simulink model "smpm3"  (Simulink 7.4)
settings: Solver=ode15s  StartTime=0.0  StopTime=0.05  RelTol=1e-3

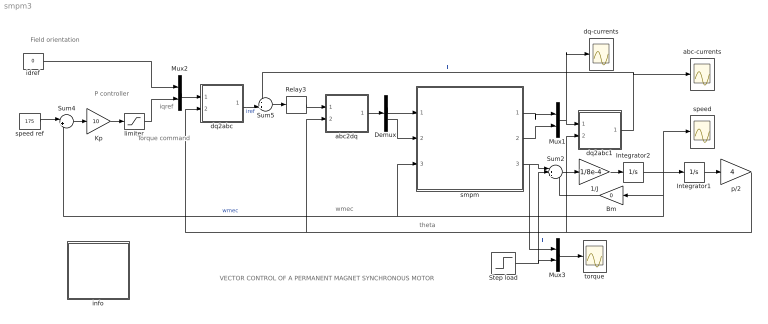
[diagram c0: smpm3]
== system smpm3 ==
  note: VECTOR CONTROL OF A PERMANENT MAGNET SYNCHRONOUS MOTOR
  note: theta
  note: wmec
  note: iqref
  note: Field orientation
  note: Torque command
  note: P controller
  1/J : Gain  Gain=1/8e-4  ParameterDataType=sfix(16)  ParameterScaling=2^0  OutDataType=sfix(16)  OutScaling=2^0
  Bm : Gain  Gain=0  ParameterDataType=sfix(16)  ParameterScaling=2^0  OutDataType=sfix(16)  OutScaling=2^0
  Demux : Demux  Outputs=2
  Integrator1 : Integrator
  Integrator2 : Integrator
  Kp : Gain  Gain=10  ParameterDataType=sfix(16)  ParameterScaling=2^0  OutDataType=sfix(16)  OutScaling=2^0
  Mux1 : Mux  Inputs=2
  Mux2 : Mux  Inputs=2
  Mux3 : Mux  Inputs=2
  Relay3 : Relay  OnSwitchValue=0.1  OffSwitchValue=-0.1  OnOutputValue=155  OffOutputValue=-155  OutDataType=sfix(16)  OutScaling=2^0
  Step load : Step  Time=0.03  Before=3  SampleTime=0
  Sum2 : Sum  Inputs=|+--  OutDataType=sfix(16)  OutScaling=2^0
  Sum4 : Sum  Inputs=|+-  OutDataType=sfix(16)  OutScaling=2^0
  Sum5 : Sum  Inputs=-+|  OutDataType=sfix(16)  OutScaling=2^0
  abc-currents : Scope
  abc2dq : Subsystem
  dq-currents : Scope
  dq2abc : Subsystem
  dq2abc1 : Subsystem
  idref : Constant  Value=0  OutDataType=sfix(16)  OutScaling=2^0
  info : Subsystem
  limiter : Saturate  UpperLimit=10  LowerLimit=-10
  p/2 : Gain  Gain=4  ParameterDataType=sfix(16)  ParameterScaling=2^0  OutDataType=sfix(16)  OutScaling=2^0
  smpm : Subsystem  mask{Ra=2.875, Lq=8.5e-3, Ld=8.5e-3, phim=0.175, p=8}
      mask prompts: Ra "Armature resistance [Ohm]"; Lq "Q_axis inductance [H]"; Ld "D_axis inductance [H}"; phim "PM flux [Wb]"; p "Number of poles"
      mask help: Model of PM synchronous machine in rotor frame.
  speed : Scope
  speed ref : Constant  Value=175  OutDataType=sfix(16)  OutScaling=2^0
  torque : Scope
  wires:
  Sum2/1 -> 1/J/1
  1/J/1 -> Integrator2/1
  Integrator2/1 -> speed/1, Bm/1, smpm/3(wmec), Sum4/2, Integrator1/1  "wmec"
  Bm/1 -> Sum2/3
  speed ref/1 -> Sum4/1
  Sum4/1 -> Kp/1
  limiter/1 -> Mux2/2
  idref/1 -> Mux2/1
  Mux1/1 -> dq2abc1/1(dq), dq-currents/1
  smpm/1(id) -> Mux1/1
  smpm/2(iq) -> Mux1/2
  dq2abc/1(abc) -> Sum5/2  "iref"
  dq2abc1/1(abc) -> Sum5/1, abc-currents/1  "i"
  Sum5/1 -> Relay3/1
  Relay3/1 -> abc2dq/1(abc)
  abc2dq/1(dq) -> Demux/1
  Demux/1 -> smpm/1(vd)
  Integrator1/1 -> p/2/1
  p/2/1 -> dq2abc/2(theta), abc2dq/2(theta), dq2abc1/2(theta)
  smpm/3(Te) -> Sum2/1, Mux3/1
  Step load/1 -> Sum2/2, Mux3/2  "Tl"
  Mux3/1 -> torque/1
  Demux/2 -> smpm/2(vq)
  Mux2/1 -> dq2abc/1(dq)
  Kp/1 -> limiter/1

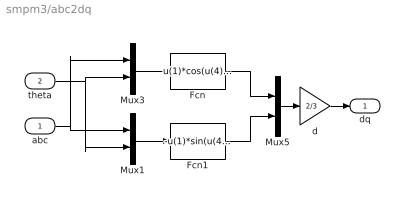
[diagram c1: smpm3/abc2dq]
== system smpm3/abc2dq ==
  abc : Inport  OutDataType=sfix(16)  OutScaling=2^0
  theta : Inport  Port=2  OutDataType=sfix(16)  OutScaling=2^0
  Fcn : Fcn  Expr=u(1)*cos(u(4))+u(2)*cos(u(4)-2*pi/3)+u(3)*cos(u(4)+2*pi/3)
  Fcn1 : Fcn  Expr=-u(1)*sin(u(4))-u(2)*sin(u(4)-2*pi/3)-u(3)*sin(u(4)+2*pi/3)
  Mux1 : Mux  Inputs=2
  Mux3 : Mux  Inputs=2
  Mux5 : Mux  Inputs=2
  d : Gain  Gain=2/3  ParameterDataType=sfix(16)  ParameterScaling=2^0  OutDataType=sfix(16)  OutScaling=2^0
  dq : Outport
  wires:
  Mux3/1 -> Fcn/1
  Fcn/1 -> Mux5/1
  Mux5/1 -> d/1
  Mux1/1 -> Fcn1/1
  Fcn1/1 -> Mux5/2
  abc/1 -> Mux1/1, Mux3/1
  theta/1 -> Mux3/2, Mux1/2
  d/1 -> dq/1

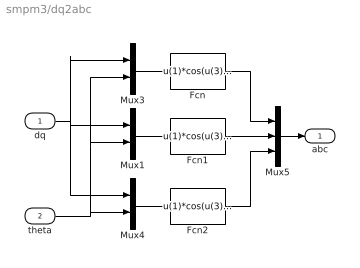
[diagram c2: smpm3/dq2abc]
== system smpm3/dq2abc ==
  dq : Inport  OutDataType=sfix(16)  OutScaling=2^0
  theta : Inport  Port=2  OutDataType=sfix(16)  OutScaling=2^0
  Fcn : Fcn  Expr=u(1)*cos(u(3))-u(2)*sin(u(3))
  Fcn1 : Fcn  Expr=u(1)*cos(u(3)-2*pi/3)-u(2)*sin(u(3)-2*pi/3)
  Fcn2 : Fcn  Expr=u(1)*cos(u(3)+2*pi/3)-u(2)*sin(u(3)+2*pi/3)
  Mux1 : Mux  Inputs=2
  Mux3 : Mux  Inputs=2
  Mux4 : Mux  Inputs=2
  Mux5 : Mux  Inputs=3
  abc : Outport
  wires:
  Mux3/1 -> Fcn/1
  Mux4/1 -> Fcn2/1
  dq/1 -> Mux3/1, Mux4/1, Mux1/1
  Fcn/1 -> Mux5/1
  Mux5/1 -> abc/1
  Mux1/1 -> Fcn1/1
  Fcn1/1 -> Mux5/2
  Fcn2/1 -> Mux5/3
  theta/1 -> Mux4/2, Mux3/2, Mux1/2

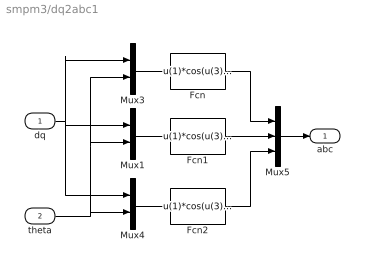
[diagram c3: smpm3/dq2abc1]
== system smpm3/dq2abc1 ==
  dq : Inport  OutDataType=sfix(16)  OutScaling=2^0
  theta : Inport  Port=2  OutDataType=sfix(16)  OutScaling=2^0
  Fcn : Fcn  Expr=u(1)*cos(u(3))-u(2)*sin(u(3))
  Fcn1 : Fcn  Expr=u(1)*cos(u(3)-2*pi/3)-u(2)*sin(u(3)-2*pi/3)
  Fcn2 : Fcn  Expr=u(1)*cos(u(3)+2*pi/3)-u(2)*sin(u(3)+2*pi/3)
  Mux1 : Mux  Inputs=2
  Mux3 : Mux  Inputs=2
  Mux4 : Mux  Inputs=2
  Mux5 : Mux  Inputs=3
  abc : Outport
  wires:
  theta/1 -> Mux1/2, Mux3/2, Mux4/2
  Fcn2/1 -> Mux5/3
  Fcn1/1 -> Mux5/2
  Mux1/1 -> Fcn1/1
  Mux5/1 -> abc/1
  Fcn/1 -> Mux5/1
  Mux4/1 -> Fcn2/1
  Mux3/1 -> Fcn/1
  dq/1 -> Mux3/1, Mux1/1, Mux4/1

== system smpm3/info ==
  note: A three-phase motor rated 1.1 KW, 220 V, 3000 rpm is fed by a PWM inverter. In this demo, the whole system is buildt entirely with standard Simulink blocks (without resort to blocksets). The initial load torque is set at the nominal value (3 N.m) and steps down to 1 N.m at t=0.03s. Two control loops are used: the inner loop regulates the currents and the outer loop controls the speed. Field orientation is obtained by setting id_ref to zero. The torque command iq_ref is derived from the speed controller.
  note: This demonstration illustrates the use of the PMSM in a closed-loop speed and current control on a 1.1 kW 3000 rpm industrial motor.
  note: (adapted from Power System Blockset demo)
  note: Circuit Description

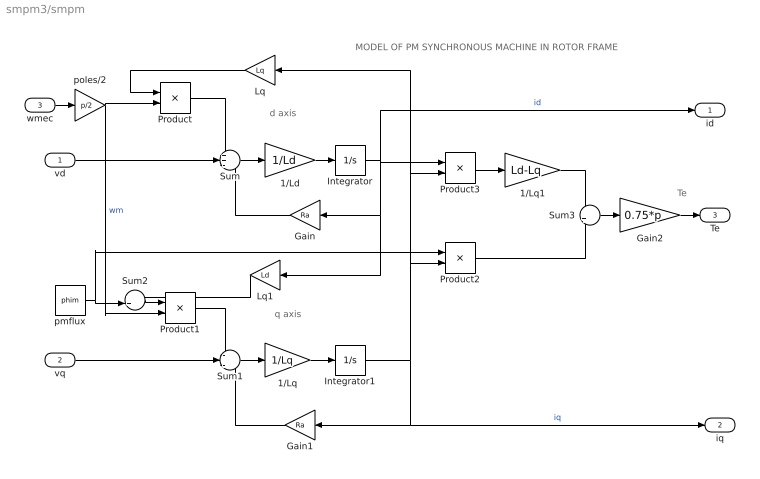
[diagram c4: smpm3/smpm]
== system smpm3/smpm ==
  note: q axis
  note: d axis
  note: Te
  note: MODEL OF PM SYNCHRONOUS MACHINE IN ROTOR FRAME
  vd : Inport  OutDataType=sfix(16)  OutScaling=2^0
  vq : Inport  Port=2  OutDataType=sfix(16)  OutScaling=2^0
  wmec : Inport  Port=3  OutDataType=sfix(16)  OutScaling=2^0
  1/Ld : Gain  Gain=1/Ld  ParameterDataType=sfix(16)  ParameterScaling=2^0  OutDataType=sfix(16)  OutScaling=2^0
  1/Lq : Gain  Gain=1/Lq  ParameterDataType=sfix(16)  ParameterScaling=2^0  OutDataType=sfix(16)  OutScaling=2^0
  1/Lq1 : Gain  Gain=Ld-Lq  ParameterDataType=sfix(16)  ParameterScaling=2^0  OutDataType=sfix(16)  OutScaling=2^0
  Gain : Gain  Gain=Ra  ParameterDataType=sfix(16)  ParameterScaling=2^0  OutDataType=sfix(16)  OutScaling=2^0
  Gain1 : Gain  Gain=Ra  ParameterDataType=sfix(16)  ParameterScaling=2^0  OutDataType=sfix(16)  OutScaling=2^0
  Gain2 : Gain  Gain=0.75*p  ParameterDataType=sfix(16)  ParameterScaling=2^0  OutDataType=sfix(16)  OutScaling=2^0
  Integrator : Integrator
  Integrator1 : Integrator
  Lq : Gain  Gain=Lq  ParameterDataType=sfix(16)  ParameterScaling=2^0  OutDataType=sfix(16)  OutScaling=2^0
  Lq1 : Gain  Gain=Ld  ParameterDataType=sfix(16)  ParameterScaling=2^0  OutDataType=sfix(16)  OutScaling=2^0
  Product{,1..3} (4 alike) : Product  OutDataType=sfix(16)  OutScaling=2^0
  Sum : Sum  Inputs=++-  OutDataType=sfix(16)  OutScaling=2^0
  Sum1 : Sum  Inputs=-+-  OutDataType=sfix(16)  OutScaling=2^0
  Sum2 : Sum  Inputs=++|  OutDataType=sfix(16)  OutScaling=2^0
  Sum3 : Sum  OutDataType=sfix(16)  OutScaling=2^0
  pmflux : Constant  Value=phim  OutDataType=sfix(16)  OutScaling=2^0
  poles/2 : Gain  Gain=p/2  ParameterDataType=sfix(16)  ParameterScaling=2^0  OutDataType=sfix(16)  OutScaling=2^0
  id : Outport
  iq : Outport  Port=2
  Te : Outport  Port=3
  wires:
  Gain/1 -> Sum/3
  vq/1 -> Sum1/2
  Gain1/1 -> Sum1/3
  Integrator/1 -> Gain/1, Lq1/1, Product3/1, id/1  "id"
  Product1/1 -> Sum1/1
  Product/1 -> Sum/1
  Lq/1 -> Product/1
  vd/1 -> Sum/2
  Sum1/1 -> 1/Lq/1
  Sum/1 -> 1/Ld/1
  Sum3/1 -> Gain2/1
  Gain2/1 -> Te/1
  wmec/1 -> poles/2/1
  poles/2/1 -> Product/2, Product1/2  "wm"
  1/Ld/1 -> Integrator/1
  1/Lq/1 -> Integrator1/1
  Integrator1/1 -> Product2/2, Product3/2, Lq/1, Gain1/1, iq/1  "iq"
  Sum2/1 -> Product1/1
  pmflux/1 -> Sum2/2, Product2/1
  Product3/1 -> 1/Lq1/1
  Product2/1 -> Sum3/2
  1/Lq1/1 -> Sum3/1
  Lq1/1 -> Sum2/1
